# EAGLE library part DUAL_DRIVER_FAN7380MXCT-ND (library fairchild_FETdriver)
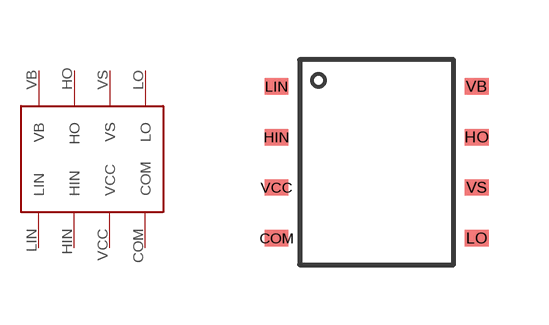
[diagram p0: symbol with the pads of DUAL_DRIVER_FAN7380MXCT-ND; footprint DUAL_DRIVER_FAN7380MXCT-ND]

Designator prefix -

## DUAL_DRIVER_FAN7380MXCT-ND  [DUAL_DRIVER_FAN7380MXCT-ND]
COM  COM
HIN  HIN
HO  HO
LIN  LIN
LO  LO
VB  VB
VCC  VCC
VS  VS

## Footprint DUAL_DRIVER_FAN7380MXCT-ND (pad centres in mm)
smd 0.6 x 0.41: COM -2.5,-1.9; HIN -2.5,0.63; HO 2.5,0.63; LIN -2.5,1.9; LO 2.5,-1.9; VB 2.5,1.9; VCC -2.5,-0.63; VS 2.5,-0.63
